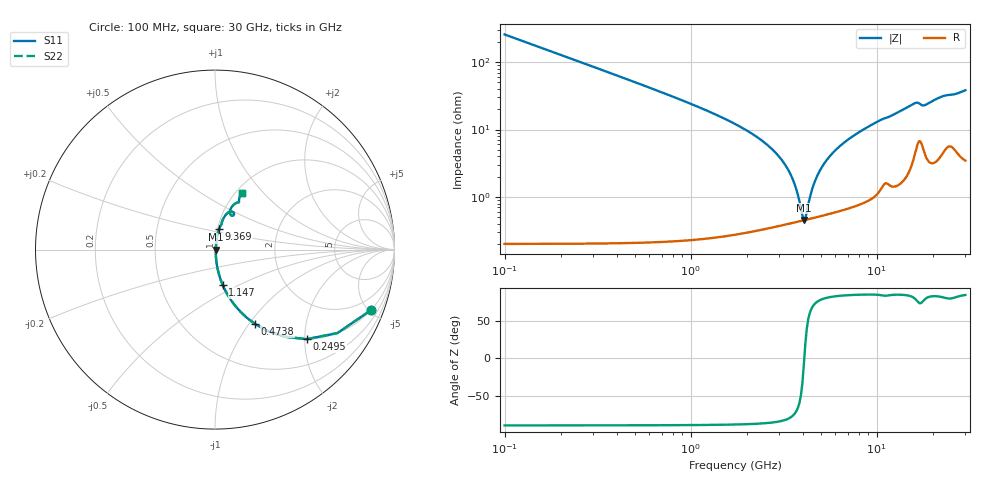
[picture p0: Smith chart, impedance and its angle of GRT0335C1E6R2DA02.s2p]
!Murata Part Number: GRT0335C1E6R2DA02
!These Parameters are Measured in Series Mode Connection
!Data Generated on Jun 19, 2026
!  o--ll--o
!Port1  Port2
!  o------o
!Operation Temp=25[degC], DC Bias Voltage=0[V]
!Freq. Start=100[MHz] Stop=30[GHz] 401[Steps]
# Hz S RI R 50
!Freq.(Hz) S11(Real) S11(Imag) S21(Real) S21(Imag) S12(Real) S12(Imag) S22(Real) S22(Imag)
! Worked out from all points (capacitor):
!   401 points, 100 MHz to 30 GHz, reference 50 ohm
!   read as one part in series: C = 6.2 pF near 249.5 MHz
!   lowest |Z| = 456 mohm at 4.062 GHz (marker M1)
!   series resonance near 4.084 GHz, so ESL is about 240 pH
!   S11 on the Smith chart (normalised r, x): 100 MHz: 1.00, -5.13; 249.5 MHz: 1.00, -2.05; 473.8 MHz: 1.00, -1.07; 1.147 GHz: 1.00, -0.41; 9.369 GHz: 1.02, +0.23; 30 GHz: 1.07, +0.76
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1e8  0.8679 -0.3382  0.1321 0.3382  0.1321 0.3382  0.8679 -0.3382
2.495e8  0.5123 -0.4989  0.4877 0.4989  0.4877 0.4989  0.5123 -0.4989
4.7375e8  0.223 -0.4143  0.777 0.4143  0.777 0.4143  0.223 -0.4143
6.98e8  0.1144 -0.3152  0.8856 0.3152  0.8856 0.3152  0.1144 -0.3152
1.1465e9  0.0427 -0.1965  0.9573 0.1965  0.9573 0.1965  0.0427 -0.1965
3.16475e9  0.00485 -0.0318  0.9952 0.0318  0.9952 0.0318  0.00485 -0.0318
3.5385e9  0.00443 -0.0177  0.9956 0.0177  0.9956 0.0177  0.00443 -0.0177
3.91225e9  0.00441 -0.00528  0.9956 0.00528  0.9956 0.00528  0.00441 -0.00528
4.06175e9  0.00449 -0.000658  0.9955 0.000658  0.9955 0.000658  0.00449 -0.000658
4.21125e9  0.00462 0.00379  0.9954 -0.00379  0.9954 -0.00379  0.00462 0.00379
4.65975e9  0.00519 0.0163  0.9948 -0.0163  0.9948 -0.0163  0.00519 0.0163
5.10825e9  0.00601 0.0277  0.994 -0.0277  0.994 -0.0277  0.00601 0.0277
5.781e9  0.00762 0.0434  0.9924 -0.0434  0.9924 -0.0434  0.00762 0.0434
6.678e9  0.0103 0.0625  0.9897 -0.0625  0.9897 -0.0625  0.0103 0.0625
9.369e9  0.0223 0.1129  0.9777 -0.1129  0.9777 -0.1129  0.0223 0.1129
1.01165e10  0.0273 0.1258  0.9727 -0.1258  0.9727 -0.1258  0.0273 0.1258
1.505e10  0.0678 0.2018  0.9322 -0.2018  0.9322 -0.2018  0.0678 0.2018
1.632075e10  0.0976 0.2099  0.9024 -0.2099  0.9024 -0.2099  0.0976 0.2099
1.781575e10  0.089 0.1918  0.911 -0.1918  0.911 -0.1918  0.089 0.1918
2.005825e10  0.0904 0.2332  0.9096 -0.2332  0.9096 -0.2332  0.0904 0.2332
2.50665e10  0.1339 0.2648  0.8661 -0.2648  0.8661 -0.2648  0.1339 0.2648
3e10  0.1489 0.3134  0.8511 -0.3134  0.8511 -0.3134  0.1489 0.3134
